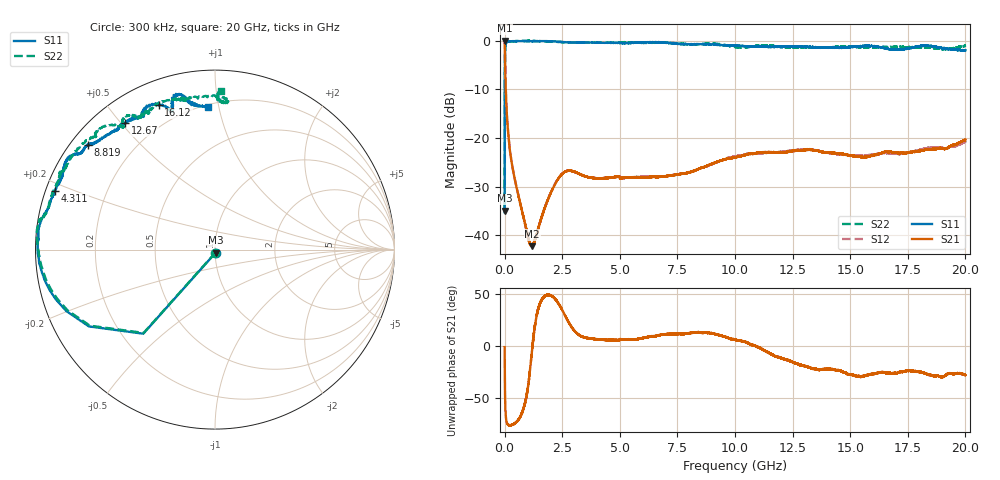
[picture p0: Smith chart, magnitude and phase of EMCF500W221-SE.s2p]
!EMCF500W221
!Johanson Technology Inc.
!www.johansontechnology.com
!Test Board Conditions:
!Substrate Type  RO4350B
!Substrate Thickness  6.6 mil
!Substrate Dk  3.66
!TL Type: GCPW
!TL Trace Width  13 mil
!TL Gap  7.5 mil
!PART MODE SINGLE ENDED (AKA BYPASS)
!DUT TOPOLOGY	SERIES-SHUNT
# MHz S  dB  R 50
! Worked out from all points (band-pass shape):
!   20001 points, 300 kHz to 20 GHz, reference 50 ohm
!   highest |S21| = 0.02 dB at 300 kHz (marker M1); lowest = -42.2 dB at 1.197 GHz (marker M2)
!   |S21| within 3 dB of the highest: start of sweep to 15.62 MHz
!   lowest |S11| = -35.0 dB at 300 kHz (marker M3), VSWR 1.04, Z = 50.3 - j1.77 ohm
!   |S11| at or under -10 dB: start of sweep to 5.474 MHz
!   |S22| runs from -35.5 to 0.0 dB; largest |S21 - S12| = 0.0052
!   S11 on the Smith chart (normalised r, x): 300 kHz: 1.01, -0.04; 4.311 GHz: 0.03, +0.18; 8.819 GHz: 0.05, +0.36; 12.67 GHz: 0.09, +0.51; 16.12 GHz: 0.11, +0.68; 20 GHz: 0.21, +0.93
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0.3  -34.97 -79.8  0.02 -1.4  0.04 -1.4  -35.51 -82.5
101.298  -0.29 -171.1  -15.54 -74.4  -15.49 -74.4  -0.36 -171.0
116.298  -0.24 -172.4  -16.65 -75.1  -16.60 -75.2  -0.32 -172.3
224.297  -0.14 -176.9  -22.34 -76.5  -22.30 -76.6  -0.21 -177.3
407.294  -0.11 -179.7  -27.64 -75.4  -27.65 -75.5  -0.12 179.2
1014.285  -0.10 177.6  -40.33 -39.8  -40.47 -39.5  -0.04 172.0
1197.282  -0.12 176.6  -42.23 -3.8  -42.20 -3.2  -0.07 171.0
1867.272  -0.11 172.4  -32.81 48.8  -32.71 48.7  -0.19 169.7
2346.265  -0.22 168.8  -28.26 40.2  -28.22 39.9  -0.27 168.7
2749.259  -0.34 166.8  -26.73 23.7  -26.73 23.3  -0.36 166.9
3334.25  -0.38 164.8  -27.56 9.0  -27.59 9.0  -0.35 162.8
4311.235  -0.45 159.9  -28.27 5.6  -28.24 5.6  -0.41 156.6
6667.2  -0.32 148.0  -28.01 9.9  -27.98 9.7  -0.42 147.6
8819.168  -0.75 140.5  -25.66 12.2  -25.73 12.2  -0.60 135.2
10000.15  -1.07 136.4  -23.98 5.8  -23.76 6.0  -1.30 127.3
12668.11  -1.28 125.4  -22.61 -17.4  -22.49 -17.2  -1.35 118.7
13334.1  -1.34 121.5  -22.46 -21.9  -22.32 -22.3  -1.41 116.0
16118.06  -1.28 111.2  -23.45 -26.8  -23.36 -28.6  -1.41 101.6
16667.05  -1.76 107.9  -22.87 -26.2  -23.18 -27.6  -1.31 103.9
17247.04  -1.80 106.8  -23.06 -25.1  -23.17 -24.1  -1.33 102.5
18609.02  -1.18 102.0  -22.28 -29.2  -21.98 -30.0  -1.55 85.9
20000  -1.98 93.0  -20.36 -28.3  -20.76 -27.2  -1.08 87.9
